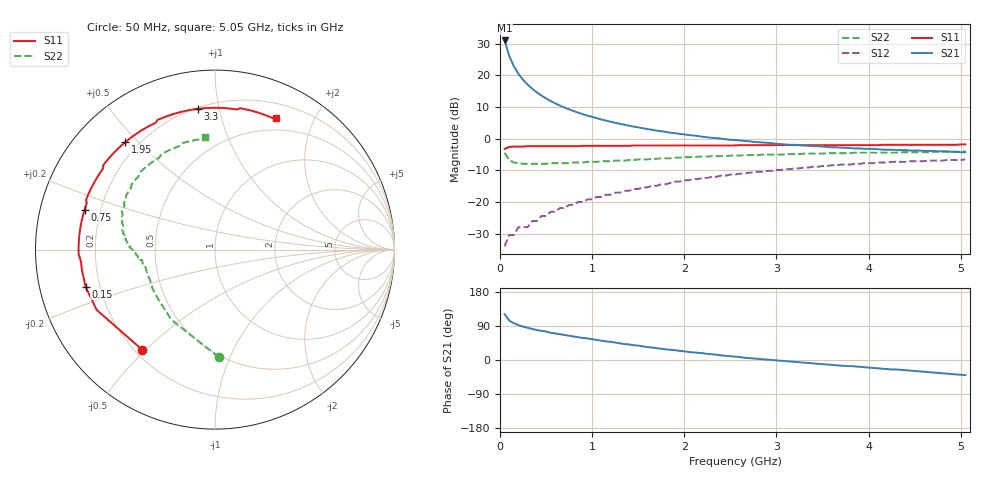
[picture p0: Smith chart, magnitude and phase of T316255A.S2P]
!AT-31625
!S-PARAMETERS at Vce=4.8 V  Ic=50 mA.  LAST UPDATED 08-05-96
# ghz s ma r 50
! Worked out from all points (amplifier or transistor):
!   101 points, 50 MHz to 5.05 GHz, reference 50 ohm
!   highest |S21| = 31.0 dB at 50 MHz (marker M1)
!   |S21| within 3 dB of that: start of sweep to 80.75 MHz
!   unconditionally stable (mu >= 1): 579.9 MHz to 637.6 MHz; 657.4 MHz to 1.434 GHz
!   at 850 MHz: K = 1.02, MAG = 13.2 dB, |S12| = -20.0 dB
!   at 2.55 GHz: K = 0.94, MSG = 5.5 dB, |S12| = -11.4 dB
!   at 5.05 GHz: K = 0.93, MSG = 1.1 dB, |S12| = -6.6 dB
!   S11 on the Smith chart (normalised r, x): 50 MHz: 0.23, -0.49; 150 MHz: 0.15, -0.14; 750 MHz: 0.14, +0.15; 1.95 GHz: 0.15, +0.46; 3.3 GHz: 0.21, +0.86; 5.05 GHz: 0.35, +1.51
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0.05  0.69 -126.0  35.63 121.0  0.02 43.0  0.6 -88.0
0.1  0.74 -153.0  20.32 104.0  0.03 38.0  0.46 -122.0
0.15  0.75 -164.0  13.94 97.0  0.03 40.0  0.42 -139.0
0.2  0.75 -171.0  10.59 92.0  0.04 44.0  0.41 -148.0
0.25  0.75 -175.0  8.53 88.0  0.04 47.0  0.4 -154.0
0.3  0.76 -178.0  7.13 85.0  0.04 50.0  0.4 -158.0
0.35  0.76 179.0  6.14 82.0  0.05 52.0  0.4 -161.0
0.4  0.76 176.0  5.38 79.0  0.05 54.0  0.4 -163.0
0.45  0.76 174.0  4.79 77.0  0.06 56.0  0.4 -165.0
0.55  0.76 170.0  3.93 72.0  0.07 58.0  0.41 -168.0
0.65  0.76 167.0  3.33 68.0  0.08 59.0  0.41 -170.0
0.75  0.76 163.0  2.9 64.0  0.09 60.0  0.41 -172.0
0.9  0.77 159.0  2.43 58.0  0.1 60.0  0.42 -174.0
1.1  0.77 153.0  2.01 51.0  0.12 59.0  0.44 -176.0
1.35  0.77 146.0  1.66 42.0  0.15 57.0  0.45 -179.0
1.75  0.78 135.0  1.31 30.0  0.19 52.0  0.49 176.0
1.95  0.78 130.0  1.19 24.0  0.21 49.0  0.5 173.0
2.55  0.78 115.0  0.95 9.0  0.27 39.0  0.54 163.0
3.3  0.79 97.0  0.78 -7.0  0.35 26.0  0.58 149.0
3.4  0.79 95.0  0.76 -9.0  0.36 23.0  0.58 146.0
4.25  0.8 79.0  0.67 -25.0  0.43 5.0  0.6 122.0
5.05  0.81 65.0  0.61 -40.0  0.47 -13.0  0.63 95.0
